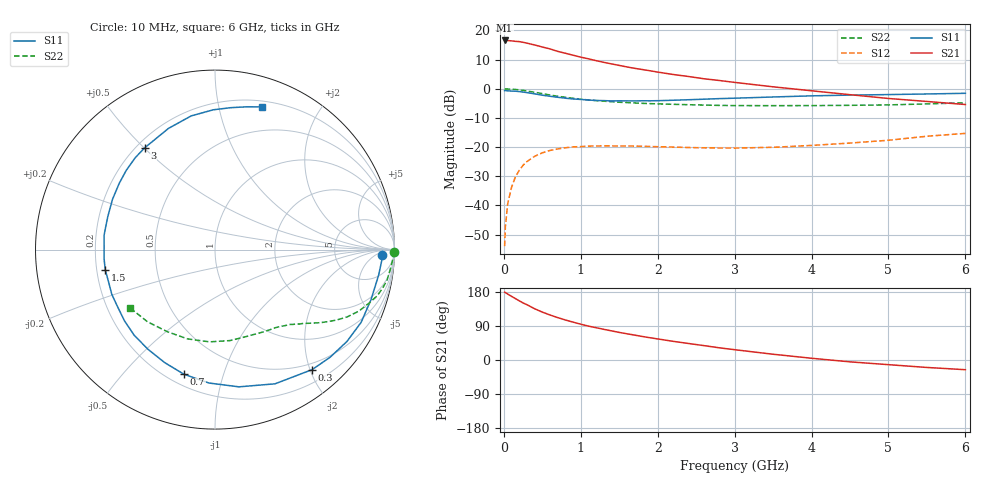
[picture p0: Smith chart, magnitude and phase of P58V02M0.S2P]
! SIEMENS Small Signal Semiconductors
! BFP183
! Si NPN RF Bipolar Junction Transistor in SOT143
! VCE = 8 V  IC = 2 mA
! Common Emitter S-Parameters:  March  1996
# GHz  S  MA  R  50
!  f  S11  S21  S12  S22
! GHz  MAG  ANG  MAG  ANG  MAG  ANG  MAG  ANG
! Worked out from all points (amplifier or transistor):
!   36 points, 10 MHz to 6 GHz, reference 50 ohm
!   highest |S21| = 16.6 dB at 10 MHz (marker M1)
!   |S21| within 3 dB of that: start of sweep to 612.5 MHz
!   unconditionally stable (mu >= 1): 2.167 GHz to 5.854 GHz
!   at 250 MHz: K = 0.12, MSG = 21.1 dB, |S12| = -26.2 dB
!   at 1.4 GHz: K = 0.66, MSG = 14.1 dB, |S12| = -19.6 dB
!   at 6 GHz: K = 0.97, MSG = 4.9 dB, |S12| = -15.3 dB
!   S11 on the Smith chart (normalised r, x): 10 MHz: 24, -10; 300 MHz: 0.40, -2.03; 700 MHz: 0.26, -0.75; 1.5 GHz: 0.24, -0.09; 3 GHz: 0.23, +0.50; 6 GHz: 0.25, +1.35
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0.01  0.932 -1.7  6.741 179.0  0.002 87.6  0.9974 -0.7
0.02  0.9314 -3.6  6.737 178.1  0.0043 81.9  0.9926 -1.3
0.05  0.9228 -8.8  6.712 174.0  0.0107 85.2  0.9913 -3.3
0.1  0.913 -17.8  6.633 168.0  0.0204 79.6  0.982 -6.6
0.2  0.8957 -34.9  6.441 156.2  0.0399 70.2  0.9587 -12.9
0.25  0.878 -43.1  6.261 150.6  0.0487 65.9  0.9395 -15.9
0.3  0.8602 -51.0  6.059 145.9  0.0564 61.5  0.915 -18.5
0.4  0.8192 -65.9  5.642 135.3  0.0695 53.6  0.8725 -23.1
0.5  0.7762 -80.1  5.206 126.4  0.0798 46.7  0.8262 -27.0
0.6  0.7441 -92.6  4.831 118.8  0.0876 41.0  0.7826 -30.1
0.7  0.7155 -104.0  4.382 111.9  0.0931 36.1  0.7452 -32.6
0.9  0.6693 -123.8  3.763 99.9  0.1008 28.3  0.6877 -36.5
1.1  0.6416 -141.9  3.264 89.4  0.104 22.5  0.6429 -39.7
1.3  0.6267 -156.6  2.838 80.9  0.105 18.1  0.6127 -42.6
1.5  0.6218 -169.6  2.518 72.8  0.1044 15.2  0.5876 -45.2
1.8  0.6232 172.8  2.139 62.1  0.1034 12.2  0.5627 -49.3
2.2  0.636 154.0  1.759 49.3  0.1002 10.3  0.5416 -55.4
3  0.6895 124.5  1.287 27.2  0.0962 13.3  0.5149 -70.1
3.5  0.7233 111.0  1.081 15.2  0.0992 17.3  0.5138 -80.6
4.5  0.779 90.7  0.792 -4.9  0.1173 23.5  0.5204 -107.0
5.5  0.8148 77.5  0.606 -19.7  0.1535 24.5  0.5506 -133.1
6  0.8366 71.9  0.537 -25.6  0.1719 21.4  0.5744 -145.7
